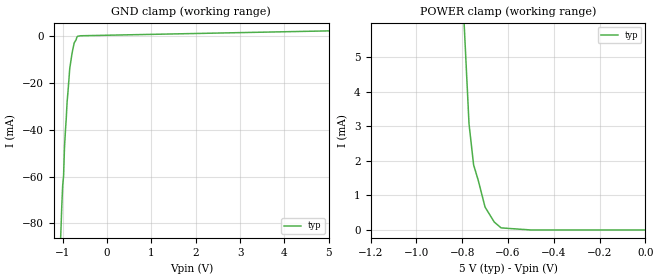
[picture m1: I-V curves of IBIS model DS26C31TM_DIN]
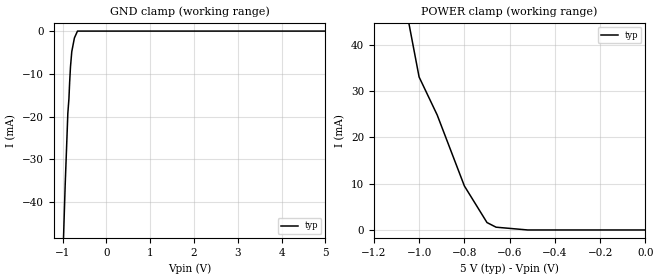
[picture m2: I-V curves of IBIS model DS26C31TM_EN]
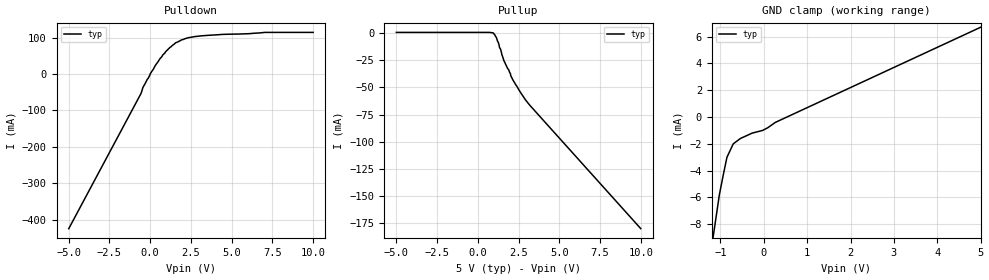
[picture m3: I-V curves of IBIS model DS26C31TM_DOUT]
|   National Semiconductor Corporation
|   Interface Products Group
|   IBIS Model of DS26C31TM
|   16L SOIC NARROW Package
[IBIS Ver]   3.2
[File name]   ds26c31tm.ibs
[File Rev]   1.1
[Date]   5/28/03
[Source]   File originated at National Semiconductor Corporation.
   Data Transmission Products group. All data based on
   Empirical Measurements(Bench).
[Notes]   All Data reused from the DS26C31 model;
   Only the pin parasitics modified;
   File created by Davor Glisic.
[Disclaimer]
(C) Copyright National Semiconductor Corporation 1994
   All rights reserved
   National Semiconductor Corporation hereby grants
the user of this IBIS model a non-exclusive, nontransferable
license to use this IBIS model under the following terms.
Before using this IBIS model, the user should read this
license.  If the user does not accept these terms,  the
IBIS model should be returned to National within 30 days.
   The user is granted this license only to use the
IBIS model and is not granted rights to sell, load, rent,
lease or license the IBIS model in whole or in part, or in
modified form to anyone other than user. User may modify
the IBIS model to suit its specific applications but rights
to derivative works and such modifications shall belong to
National.
   This IBIS model is provided on an "AS IS" basis and
National makes absolutely no warranty with respect to the
information contained herein.NATIONAL DISCLAIMS AND CUSTOMER
WAIVES ALL WARRANTIES, EXPRESS OR IMPLIED, INCLUDING
WARRANTIES OF MERCHANTABILITY OR FITNESS FOR A PARTICULAR
PURPOSE. The entire risk as to quality and performance is
with the Customer. ACCORDINGLY, IN NO EVENT SHALL THE
COMPANY BE LIABLE FOR ANY DAMAGES, WHETHER IN CONTRACT OR
TORT,INCLUDING ANY LOST PROFITS OR OTHER INCIDENTAL,
CONSEQUENTIAL, EXEMPLARY, OR PUNITIVE DAMAGES ARISING OUT
OF THE USE OR APPLICATION OF THE IBIS model provided in
this package.Further, National reserves the right to make
changes without notice to any product herein to improve
reliability, function, or design. National does not convey
any license under patent rights or any other intellectual
property rights, including those of third parties.
   National is not obligated to provide maintenance or support
for the licensed IBIS model.
Contact National at ATTN:INTERFACE APPLICATIONS/IBIS MODELS.
2900 Semiconductor Drive, M/S A2595, Santa Clara, CA 95052-8090
[Disclaimer] IBIS Open Forum disclaims all warranties. See DISCLAIM.TXT
   in vhdl.org:/pub/IBIS/models for the full disclaimer.
[Copyright]   Copyright 2003, National Semiconductor, All Rights Reserved
[Component]   DS26C31TM
[Manufacturer]  National Semiconductor Corp
[Package]
|   typ   min   max
R_pkg   50.0m   50.0m   50.0m
L_pkg   1.37nH   0.95nH   2.07nH
C_pkg   0.26pF   0.146pF   0.429pF
[Pin]   signal_name   model_name   R_pin   L_pin   C_pin
1   DIN1   DS26C31TM_DIN   50.0m   2.07nH   0.429pF
2   DOUT1+   DS26C31TM_DOUT   50.0m   1.49nH   0.306pF
3   DOUT1-   DS26C31TM_DOUT   50.0m   0.95nH   0.146pF
4   EN   DS26C31TM_EN   50.0m   0.95nH   0.152pF
5   DOUT2-   DS26C31TM_DOUT   50.0m   0.95nH   0.152pF
6   DOUT2+   DS26C31TM_DOUT   50.0m   0.95nH   0.146pF
7   DIN2   DS26C31TM_DIN   50.0m   1.49nH   0.306pF
8   GND   GND   50.0m   2.07nH   0.429pF
9   DIN3   DS26C31TM_DIN   50.0m   2.07nH   0.429pF
10   DOUT3+   DS26C31TM_DOUT   50.0m   1.49nH   0.306pF
11   DOUT3-   DS26C31TM_DOUT   50.0m   0.95nH   0.146pF
12   EN*   DS26C31TM_EN   50.0m   0.95nH   0.152pF
13   DOUT4-   DS26C31TM_DOUT   50.0m   0.95nH   0.152pF
14   DOUT4+   DS26C31TM_DOUT   50.0m   0.95nH   0.146pF
15   DIN4   DS26C31TM_DIN   50.0m   1.49nH   0.306pF
16   VCC   POWER   50.0m   2.07nH   0.429pF
[Diff_pin]   inv_pin   vdiff   tdelay_typ   tdelay_min   tdelay_max
| The '+' pin is Diff_pin and the '-' pin is the inv_pin
2   3   NA   0 0 0
6   5   NA   0 0 0
10   11   NA   0 0 0
14   13   NA   0 0 0
| Models and submodels in the file (3): DS26C31TM_DIN (Input), DS26C31TM_EN (Input), DS26C31TM_DOUT (3-state)
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|   Driver Input  MODEL
[Model]   DS26C31TM_DIN
Model_type   Input
|Signals   DIN1,DIN2,DIN3,DIN4
Vinh = 2.0
Vinl = 0.8
|   typ   min   max
C_comp   1.0pF   NA   NA
|   typ   min   max
[Temperature Range]   25.0   NA   NA
[Voltage range]   5.0V   4.5V   5.5V
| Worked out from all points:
|   GND clamp passes 1 mA (typ) near -0.69 V on its own axis
|   POWER clamp passes 1 mA (typ) near -0.71 V on its own axis
[Power_clamp]
| Note that the[POWER_clamp]voltage table is referenced to Vcc
| and is calculated using Vtable=Vcc - Vmeasured.
|   Voltage   I(typ)   I(min)   I(max)
-5V       578.3mA    NA         NA
-780mV    4.42mA     NA         NA
-770mV    3.06mA     NA         NA
-750mV    1.88mA     NA         NA
-730mV    1.44mA     NA         NA
-700mV    660uA      NA         NA
-660mV    230uA      NA         NA
-630mV    60uA       NA         NA
-500mV    0A         NA         NA
-360mV    0A         NA         NA
-200mV    0A         NA         NA
0V        0A         NA         NA
[GND_clamp]
|   Voltage   I(typ)   I(min)   I(max)
-5V       -2.222A    NA         NA
-1.04V    -83.2mA    NA         NA
-1.02V    -72.4mA    NA         NA
-1V       -63.8mA    NA         NA
-980mV    -59.8mA    NA         NA
-960mV    -47.8mA    NA         NA
-900mV    -28mA      NA         NA
-840mV    -13.6mA    NA         NA
-780mV    -6.4mA     NA         NA
-740mV    -2.8mA     NA         NA
-660mV    0A         NA         NA
5V        2.29mA     NA         NA
|   Driver Enable  MODEL
[Model]   DS26C31TM_EN
Model_type   Input
|Signals   EN,EN*
Vinh = 2.0
Vinl = 0.8
|   typ   min   max
C_comp   1.0pF   NA   NA
|   typ   min   max
[Temperature Range]   25.0   NA   NA
[Voltage range]   5.0V   4.5V   5.5V
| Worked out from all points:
|   GND clamp passes 1 mA (typ) near -0.70 V on its own axis
|   POWER clamp passes 1 mA (typ) near -0.68 V on its own axis
[GND_clamp]
|   Voltage   I(typ)   I(min)   I(max)
-5V       -1.26A     NA         NA
-1.05V    -71.6mA    NA         NA
-940mV    -35.8mA    NA         NA
-880mV    -19.2mA    NA         NA
-855mV    -15.8mA    NA         NA
-840mV    -12.2mA    NA         NA
-820mV    -8.4mA     NA         NA
-790mV    -4.8mA     NA         NA
-730mV    -1.6mA     NA         NA
-660mV    0A         NA         NA
5V        0A         NA         NA
[Power_clamp]
| Note that the[POWER_clamp]voltage table is referenced to Vcc
| and is calculated using Vtable=Vcc - Vmeasured.
|   Voltage   I(typ)   I(min)   I(max)
-5V       1.06A      NA         NA
-1.06V    48.4mA     NA         NA
-1V       33mA       NA         NA
-920mV    24.8mA     NA         NA
-800mV    9.5mA      NA         NA
-700mV    1.6mA      NA         NA
-660mV    600uA      NA         NA
-520mV    0A         NA         NA
0V        0A         NA         NA
|   Driver Output  MODEL
[Model]   DS26C31TM_DOUT
Model_type   3-state
| Signals   DOUT1+,DOUT1-,DOUT2+,DOUT2-,DOUT3+,DOUT3-,DOUT4+,DOUT4-
Vmeas = 1.3V   |Reference voltage for timing measurements
Cref = 40pF   |Timing specification test load capacitance value
Rref = 50   |Note: 100 Ohm between the two driver outputs
Vref = 1.5   |Timing specification test load voltage; GND
| variable   typ   min   max
C_comp   3.0pF   NA   NA
|   typ   min   max
[Temperature Range]   25.0   NA   NA
[Voltage range]   5.0V   4.5V   5.5V
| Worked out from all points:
|   slope of the pulldown table from 0 to 0.75 V, typ, clamps not added: 14.9 ohm
|   slope of the pullup table from 0 to 0.75 V, typ, clamps not added: 12.5 kohm
|   GND clamp passes 1 mA (typ) near -0.03 V on its own axis
[Pulldown]
|   Voltage   I(typ)   I(min)   I(max)
-5V       -425mA     NA         NA
-560mV    -53mA      NA         NA
-420mV    -34.5mA    NA         NA
-120mV    -11.5mA    NA         NA
0V        500uA      NA         NA
320mV     24mA       NA         NA
780mV     53mA       NA         NA
1.56V     86mA       NA         NA
2.3V      99.5mA     NA         NA
3.58V     106.5mA    NA         NA
7.02V     114.5mA    NA         NA
10V       114.5mA    NA         NA
[Pullup]
|   Voltage   I(typ)   I(min)   I(max)
| Note that the[Pullup]voltage table is referenced to Vcc
| and is calculated using Vtable=Vcc - Vmeasured.
-5V       600uA      NA         NA
960mV     0A         NA         NA
1.16V     -5mA       NA         NA
1.26V     -8.8mA     NA         NA
1.34V     -13.6mA    NA         NA
1.4V      -15mA      NA         NA
1.48V     -20.2mA    NA         NA
1.6V      -25.4mA    NA         NA
1.9V      -34mA      NA         NA
2.02V     -39.2mA    NA         NA
2.92V     -61.4mA    NA         NA
10V       -179.9mA   NA         NA
[GND_clamp]
|   Voltage   I(typ)   I(min)   I(max)
| Outputs in Tri-state.
-5V       -649.2mA   NA         NA
-1.18V    -9.2mA     NA         NA
-1.025V   -5.8mA     NA         NA
-850mV    -3mA       NA         NA
-705mV    -2mA       NA         NA
-540mV    -1.6mA     NA         NA
-270mV    -1.2mA     NA         NA
-30mV     -1mA       NA         NA
265mV     -400uA     NA         NA
5V        6.7mA      NA         NA
[POWER_clamp]
|   Voltage   I(typ)   I(min)   I(max)
| Note that the[POWER_clamp]voltage table is referenced to Vcc
| and is calculated using Vtable=Vcc - Vmeasured.
| Outputs in Tri-state.
-9.8V     0A         NA         NA
-5V       0A         NA         NA
0V        0A         NA         NA
4V        0A         NA         NA
5V        0A         NA         NA
[Ramp]
|   typ   min   max
dV/dt_r   4.5/0.75n   NA   NA
dV/dt_f   4.6/0.90n   NA   NA
R_load = 100Ohm | Note: This 100 Ohm is across the two driver output
